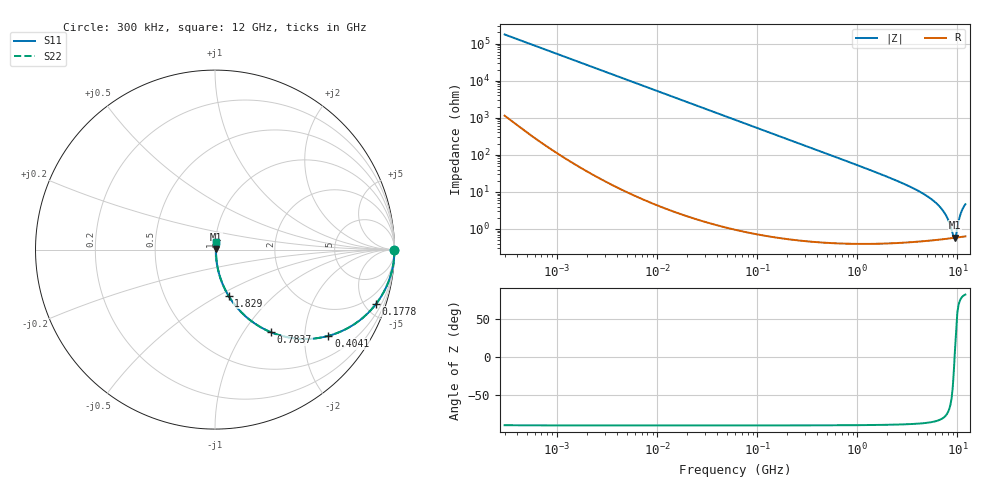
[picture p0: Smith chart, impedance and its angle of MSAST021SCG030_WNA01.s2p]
! MSAST021SCG030_WNA01  S-PARAMETER MODEL  ( General Type )
! Model Generated by TAIYO YUDEN Corporation (http://www.ty-top.com)
! Version 2.0
! TAIYO YUDEN Control No. 181101
! Copyright(c) 2015 TAIYO YUDEN CO.,LTD. All Rights Reserved.
! Product Description (link to TY-COMPAS)
! https://ds.yuden.co.jp/TYCOMPAS/or/detail?pn=MSAST021SCG030BWNA01&u=M
! Products Name : Multilayer Ceramic Capacitors
! Characteristics :
!  Capacitance : 3 pF , Rated Voltage : 25V , TCC : CG / C0G
!  Case Size : 0.25 x 0.125 / 0.0098 x 0.0049 [mm/inch] , Thickness : 0.125 / 0.0049 [mm/inch]
!  (Conditions: Temperature = 25 degC , DC Bias Current/Voltage = 0A / 0V)
! External Node Assignments :
!  1  o---| |---o  2
! GND o---------o GND
! Frequency Range : 0.3MHz  -  12000MHz  [ 401 STEP ]
# MHz S RI R 50
! Freq[MHz].  S11 Real  S11 Imag  S21 Real  S21 Imag  S12 Real  S12 Imag  S22 Real  S22 Imag
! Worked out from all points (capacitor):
!   401 points, 300 kHz to 12 GHz, reference 50 ohm
!   read as one part in series: C = 3 pF near 316.3 kHz
!   lowest |Z| = 584 mohm at 9.454 GHz (marker M1)
!   series resonance near 9.364 GHz, so ESL is about 96 pH
!   S11 on the Smith chart (normalised r, x): 300 kHz: open; 177.8 MHz: 1.01, -5.97; 404.1 MHz: 1.01, -2.62; 783.7 MHz: 1.01, -1.34; 1.829 GHz: 1.01, -0.56; 12 GHz: 1.01, +0.09
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0.3  1 -0.000565  3.96e-06 0.000565  3.96e-06 0.000565  1 -0.000565
1.769972  1 -0.00334  1.59e-05 0.00334  1.59e-05 0.00334  1 -0.00334
10.44266  0.9996 -0.0197  0.000403 0.0197  0.000403 0.0197  0.9996 -0.0197
60  0.9873 -0.1116  0.0127 0.1116  0.0127 0.1116  0.9873 -0.1116
177.7716  0.8985 -0.301  0.1015 0.301  0.1015 0.301  0.8985 -0.301
353.9943  0.6908 -0.4607  0.3092 0.4607  0.3092 0.4607  0.6908 -0.4607
404.1309  0.6315 -0.4807  0.3685 0.4807  0.3685 0.4807  0.6315 -0.4807
783.7017  0.3123 -0.4605  0.6877 0.4605  0.6877 0.4605  0.3123 -0.4605
1197.383  0.1618 -0.3638  0.8382 0.3638  0.8382 0.3638  0.1618 -0.3638
1829.429  0.0753 -0.2569  0.9247 0.2569  0.9247 0.2569  0.0753 -0.2569
2088.533  0.0584 -0.2263  0.9416 0.2263  0.9416 0.2263  0.0584 -0.2263
3944.255  0.0164 -0.1083  0.9836 0.1083  0.9836 0.1083  0.0164 -0.1083
5868.704  0.00788 -0.0541  0.9921 0.0541  0.9921 0.0541  0.00788 -0.0541
7448.838  0.00595 -0.0258  0.994 0.0258  0.994 0.0258  0.00595 -0.0258
8064.993  0.0057 -0.0167  0.9943 0.0167  0.9943 0.0167  0.0057 -0.0167
8966.534  0.00564 -0.00475  0.9944 0.00475  0.9944 0.00475  0.00564 -0.00475
9207.246  0.00567 -0.00178  0.9943 0.00178  0.9943 0.00178  0.00567 -0.00178
9454.42  0.00572 0.00103  0.9943 -0.00103  0.9943 -0.00103  0.00572 0.00103
9708.23  0.00579 0.00401  0.9942 -0.00401  0.9942 -0.00401  0.00579 0.00401
10793.46  0.00663 0.0251  0.9934 -0.0251  0.9934 -0.0251  0.00663 0.0251
11380.75  0.00739 0.0356  0.9926 -0.0356  0.9926 -0.0356  0.00739 0.0356
12000  0.00827 0.045  0.9917 -0.045  0.9917 -0.045  0.00827 0.045
